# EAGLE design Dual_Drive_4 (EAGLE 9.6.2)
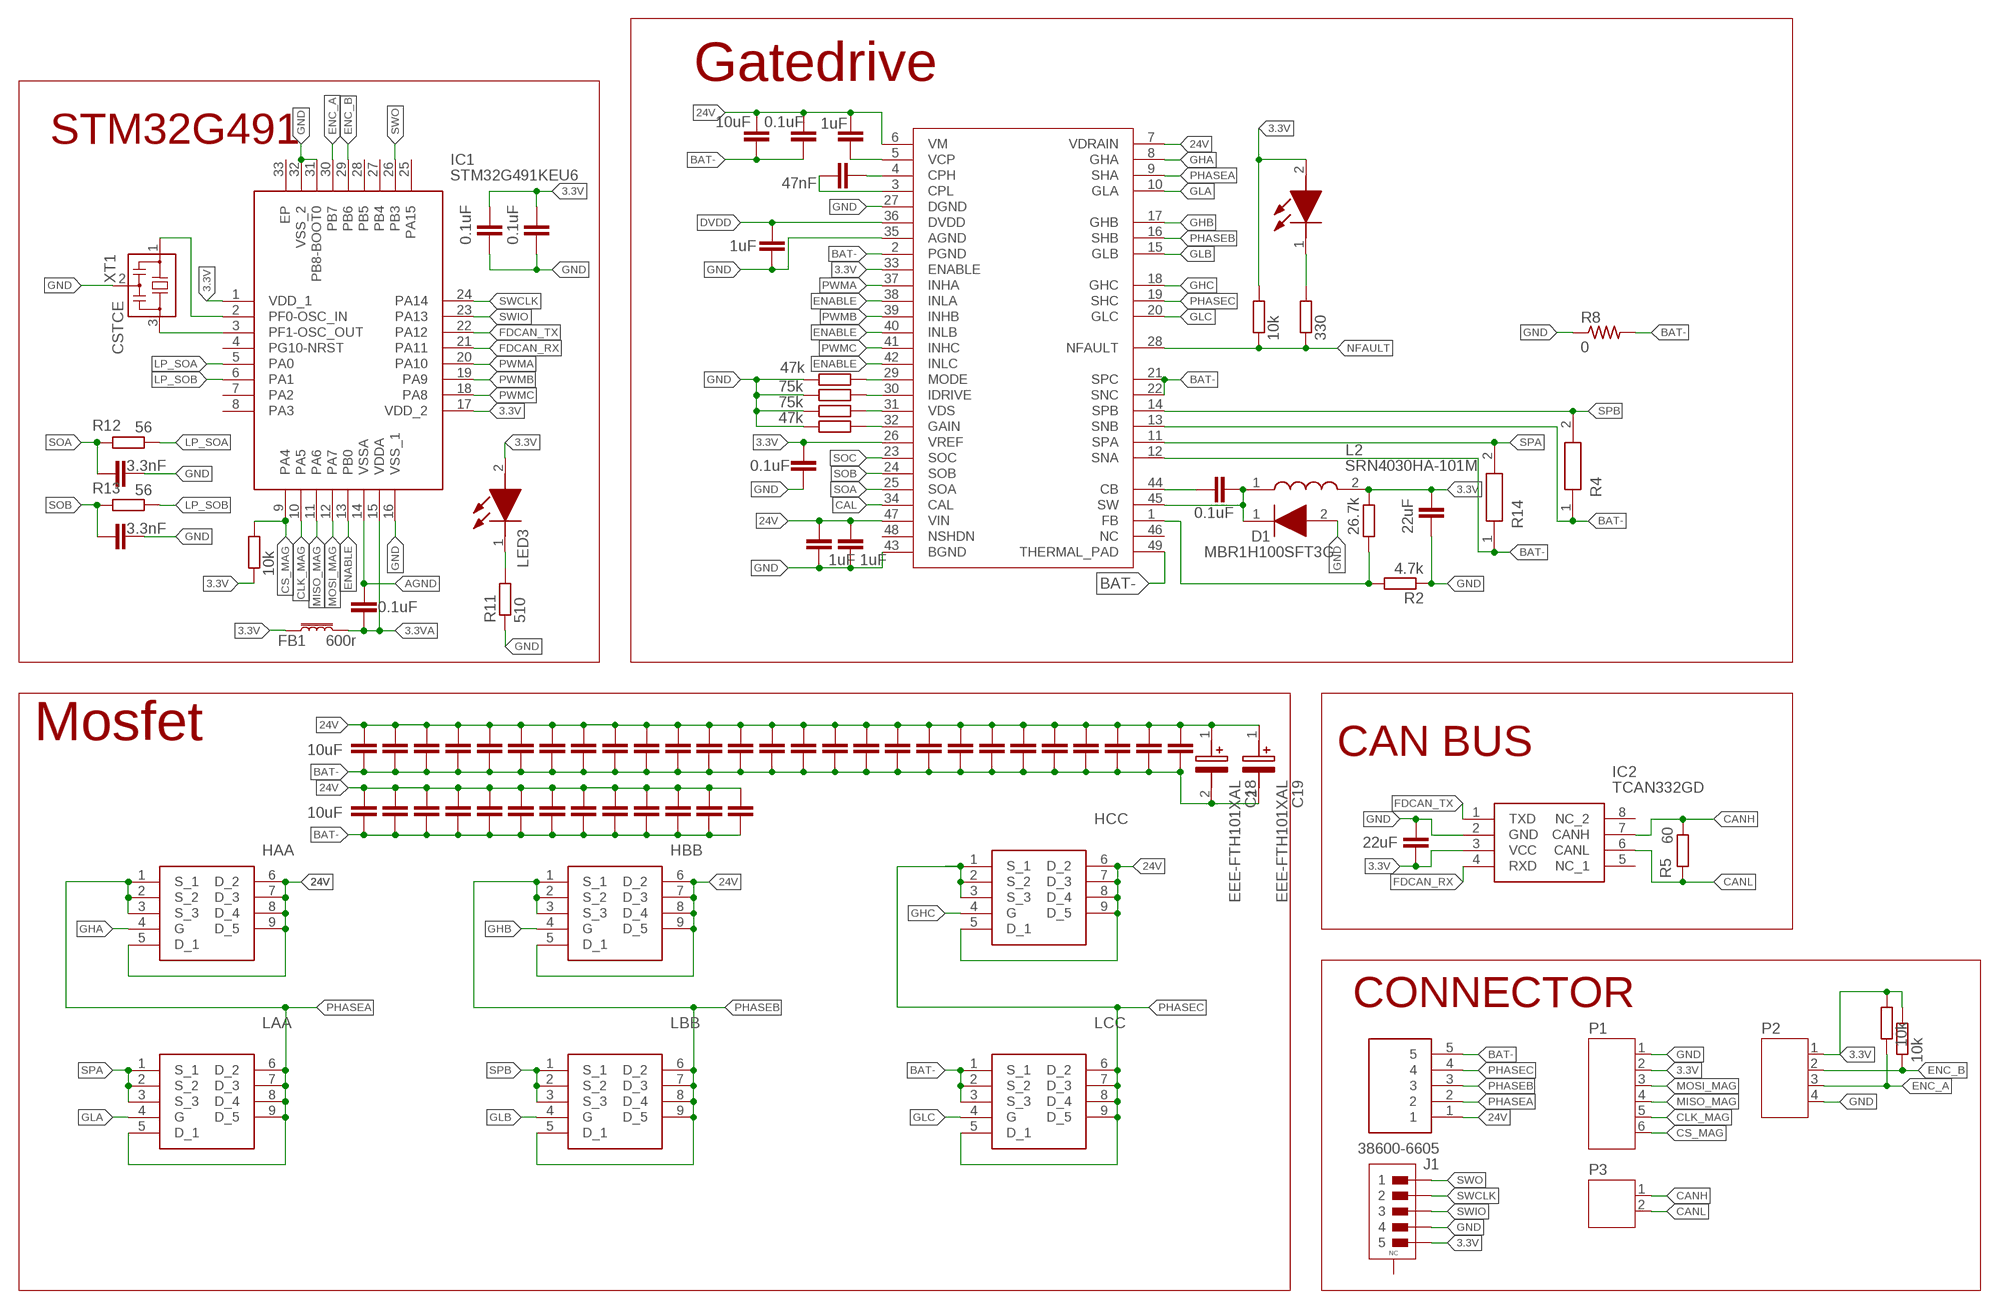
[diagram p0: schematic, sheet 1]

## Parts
C1  3.3nF  C-EUC0603  [C0603]
C2  3.3nF  C-EUC0603  [C0603]
C3  10uF  C-EU1206C1206  [C1206]
C4  22uF  C-EUC0603  [C0603]
C5  10uF  C-EU1206C1206  [C1206]
C6  10uF  C-EU1206C1206  [C1206]
C7  10uF  C-EU1206C1206  [C1206]
C8  10uF  C-EU1206C1206  [C1206]
C9  10uF  C-EU1206C1206  [C1206]
C10  0.1uF  C-EU1206C1206  [C1206]
C11  1uF  C-EUC0603  [C0603]
C12  10uF  C-EU1206C1206  [C1206]
C13  0.1uF  C-EUC0603  [C0603]
C14  1uF  C-EUC0603  [C0603]
C15  0.1uF  C-EUC0603  [C0603]
C16  10uF  C-EU1206C1206  [C1206]
C17  10uF  C-EU1206C1206  [C1206]
C18  EEE-FTH101XAL  [EEEHP1H4R7P]
C19  EEE-FTH101XAL  [EEEHP1H4R7P]
C20  10uF  C-EU1206C1206  [C1206]
C21  10uF  C-EU1206C1206  [C1206]
C22  10uF  C-EU1206C1206  [C1206]
C23  10uF  C-EU1206C1206  [C1206]
C24  10uF  C-EU1206C1206  [C1206]
C25  10uF  C-EU1206C1206  [C1206]
C26  0.1uF  C-EUC0603  [C0603]
C27  0.1uF  C-EUC0603  [C0603]
C28  10uF  C-EU1206C1206  [C1206]
C29  10uF  C-EU1206C1206  [C1206]
C30  0.1uF  C-EUC0603  [C0603]
C31  10uF  C-EU1206C1206  [C1206]
C32  10uF  C-EU1206C1206  [C1206]
C33  10uF  C-EU1206C1206  [C1206]
C34  10uF  C-EU1206C1206  [C1206]
C35  10uF  C-EU1206C1206  [C1206]
C36  10uF  C-EU1206C1206  [C1206]
C37  10uF  C-EU1206C1206  [C1206]
C38  10uF  C-EU1206C1206  [C1206]
C39  10uF  C-EU1206C1206  [C1206]
C40  10uF  C-EU1206C1206  [C1206]
C41  10uF  C-EU1206C1206  [C1206]
C42  10uF  C-EU1206C1206  [C1206]
C43  10uF  C-EU1206C1206  [C1206]
C44  10uF  C-EU1206C1206  [C1206]
C45  47nF  C-EU0805C0805  [C0805]
C46  22uF  C-EUC0603  [C0603]
C47  10uF  C-EU1206C1206  [C1206]
C48  10uF  C-EU1206C1206  [C1206]
C49  10uF  C-EU1206C1206  [C1206]
C50  10uF  C-EU1206C1206  [C1206]
C51  10uF  C-EU1206C1206  [C1206]
C52  10uF  C-EU1206C1206  [C1206]
C53  10uF  C-EU1206C1206  [C1206]
C54  10uF  C-EU1206C1206  [C1206]
C55  10uF  C-EU1206C1206  [C1206]
C56  10uF  C-EU1206C1206  [C1206]
CIN  1uF  C-EUC0603  [C0603]
CIN1  1uF  C-EUC0603  [C0603]
D1  MBR1H100SFT3G  [SODFL3616X98N]
FB1  600r  FERRITE_BEAD-0603  [0603]
HAA  TPH2R506PL,L1Q  [TPHR9003NLL1Q]
HBB  TPH2R506PL,L1Q  [TPHR9003NLL1Q]
HCC  TPH2R506PL,L1Q  [TPHR9003NLL1Q]
IC1  STM32G491KEU6  [QFN50P500X500X60-33N]
IC2  TCAN332GD  [SOIC127P600X175-8N]
IC3  DRV8323RHRGZR  [QFN50P700X700X100-49N]
J1  38600-6605  [386006605]
L2  SRN4030HA-101M  [SRN4030HA101M]
LAA  TPH2R506PL,L1Q  [TPHR9003NLL1Q]
LBB  TPH2R506PL,L1Q  [TPHR9003NLL1Q]
LCC  TPH2R506PL,L1Q  [TPHR9003NLL1Q]
LED1  LTST-C191KRKT  [LEDC1608X55N]
LED3  LTST-C191KRKT  [LEDC1608X55N]
P1  JST-PH6  [JST-PH6]
P2  JST-PH4  [JST-PH4]
P3  JST-PH2  [JST-PH2]
R1  26.7k  R-EU_R0603  [R0603]
R2  4.7k  R-EU_R0603  [R0603]
R3  47k  R-EU_R0603  [R0603]
R4  0.01  CRA2512-FZ-R010ELF  [RESC6434X90N]
R5  60  R-EU_R0603  [R0603]
R6  47k  R-EU_R0603  [R0603]
R7  75k  R-EU_R0603  [R0603]
R8  0  R-US_M1206  [M1206]
R10  75k  R-EU_R0603  [R0603]
R11  510  R-EU_R0603  [R0603]
R12  56  R-EU_R0603  [R0603]
R13  56  R-EU_R0603  [R0603]
R14  0.01  CRA2512-FZ-R010ELF  [RESC6434X90N]
RPULL  10k  R-EU_R0603  [R0603]
RPULL1  330  R-EU_R0603  [R0603]
RPULL2  10k  R-EU_R0603  [R0603]
RPULL3  10k  R-EU_R0603  [R0603]
RPULL4  10k  R-EU_R0603  [R0603]
U$3  CON-JST-PH2.0-5PIN-SMD  [CON-JST-PH2.0-5PIN-SMD]
XT1  CSTCE  [CSTCE]

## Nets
3.3V: C4.2 C15.1 C26.1 C27.1 C46.1 FB1.1 IC1.1(VDD_1) IC1.17(VDD_2) IC2.3(VCC) IC3.26(VREF) IC3.33(ENABLE) L2.2 LED1.2(A) LED3.2(A) P1.2 P2.1 R1.2 RPULL2.1 RPULL3.2 RPULL4.2 RPULL.2 U$3.5
3.3VA: C30.1 FB1.2 IC1.15(VDDA)
24V: C3.1 C5.1 C6.1 C7.1 C8.1 C9.1 C10.1 C11.1 C12.1 C16.1 C17.1 C18.1(+) C19.1(+) C20.1 C21.1 C22.1 C23.1 C24.1 C25.1 C28.1 C29.1 C31.1 C32.1 C33.1 C34.1 C35.1 C36.1 C37.1 C38.1 C39.1 C40.1 C41.1 C42.1 C43.1 C44.1 C47.1 C48.1 C49.1 C50.1 C51.1 C52.1 C53.1 C54.1 C55.1 C56.1 CIN1.1 CIN.1 HAA.5(D_1) HAA.6(D_2) HAA.7(D_3) HAA.8(D_4) HAA.9(D_5) HBB.5(D_1) HBB.6(D_2) HBB.7(D_3) HBB.8(D_4) HBB.9(D_5) HCC.5(D_1) HCC.6(D_2) HCC.7(D_3) HCC.8(D_4) HCC.9(D_5) IC3.6(VM) IC3.7(VDRAIN) IC3.47(VIN) J1.1
AGND: C30.2 IC1.14(VSSA)
BAT-: C3.2 C5.2 C6.2 C7.2 C8.2 C9.2 C10.2 C12.2 C16.2 C17.2 C18.2(-) C19.2(-) C20.2 C21.2 C22.2 C23.2 C24.2 C25.2 C28.2 C29.2 C31.2 C32.2 C33.2 C34.2 C35.2 C36.2 C37.2 C38.2 C39.2 C40.2 C41.2 C42.2 C43.2 C44.2 C47.2 C48.2 C49.2 C50.2 C51.2 C52.2 C53.2 C54.2 C55.2 C56.2 IC3.2(PGND) IC3.12(SNA) IC3.13(SNB) IC3.21(SPC) IC3.22(SNC) IC3.49(THERMAL_PAD) J1.5 LCC.1(S_1) LCC.2(S_2) LCC.3(S_3) R4.1 R8.2 R14.1
CAL: IC3.34(CAL)
CANH: IC2.7(CANH) P3.1 R5.1
CANL: IC2.6(CANL) P3.2 R5.2
CB: C13.1 IC3.44(CB)
CLK_MAG: IC1.10(PA5) P1.5
CPH: C45.2 IC3.4(CPH)
CPL: C45.1 IC3.3(CPL)
CS_MAG: IC1.9(PA4) P1.6 RPULL2.2
DVDD: C14.1 IC3.36(DVDD)
ENABLE: IC1.13(PB0) IC3.38(INLA) IC3.40(INLB) IC3.42(INLC)
ENC_A: IC1.30(PB7) P2.3 RPULL4.1
ENC_B: IC1.29(PB6) P2.2 RPULL3.1
FB: IC3.1(FB) R1.1 R2.2
FDCAN_RX: IC1.21(PA11) IC2.4(RXD)
FDCAN_TX: IC1.22(PA12) IC2.1(TXD)
GAIN: IC3.32(GAIN) R3.2
GHA: HAA.4(G) IC3.8(GHA)
GHB: HBB.4(G) IC3.17(GHB)
GHC: HCC.4(G) IC3.18(GHC)
GLA: IC3.10(GLA) LAA.4(G)
GLB: IC3.15(GLB) LBB.4(G)
GLC: IC3.20(GLC) LCC.4(G)
GND: C1.2 C2.2 C4.1 C14.2 C15.2 C26.2 C27.2 C46.2 CIN1.2 CIN.2 D1.2(A) IC1.16(VSS_1) IC1.31(PB8-BOOT0) IC1.32(VSS_2) IC2.2(GND) IC3.27(DGND) IC3.35(AGND) IC3.43(BGND) P1.1 P2.4 R2.1 R3.1 R6.1 R7.1 R8.1 R10.1 R11.1 U$3.4 XT1.2
IDRIVE: IC3.30(IDRIVE) R7.2
LEDFAULT: LED1.1(K) RPULL1.2
LP_SOA: IC1.5(PA0) R12.1
LP_SOB: IC1.6(PA1) R13.1
MISO_MAG: IC1.11(PA6) P1.4
MODE: IC3.29(MODE) R6.2
MOSI_MAG: IC1.12(PA7) P1.3
N$9: IC1.3(PF1-OSC_OUT) XT1.3
N$10: LED3.1(K) R11.2
N$11: IC1.2(PF0-OSC_IN) XT1.1
NFAULT: IC3.28(NFAULT) RPULL1.1 RPULL.1
PHASEA: HAA.1(S_1) HAA.2(S_2) HAA.3(S_3) IC3.9(SHA) J1.2 LAA.5(D_1) LAA.6(D_2) LAA.7(D_3) LAA.8(D_4) LAA.9(D_5)
PHASEB: HBB.1(S_1) HBB.2(S_2) HBB.3(S_3) IC3.16(SHB) J1.3 LBB.5(D_1) LBB.6(D_2) LBB.7(D_3) LBB.8(D_4) LBB.9(D_5)
PHASEC: HCC.1(S_1) HCC.2(S_2) HCC.3(S_3) IC3.19(SHC) J1.4 LCC.5(D_1) LCC.6(D_2) LCC.7(D_3) LCC.8(D_4) LCC.9(D_5)
PWMA: IC1.20(PA10) IC3.37(INHA)
PWMB: IC1.19(PA9) IC3.39(INHB)
PWMC: IC1.18(PA8) IC3.41(INHC)
SOA: C1.1 IC3.25(SOA) R12.2
SOB: C2.1 IC3.24(SOB) R13.2
SOC: IC3.23(SOC)
SPA: IC3.11(SPA) LAA.1(S_1) LAA.2(S_2) LAA.3(S_3) R14.2
SPB: IC3.14(SPB) LBB.1(S_1) LBB.2(S_2) LBB.3(S_3) R4.2
SW: C13.2 D1.1(K) IC3.45(SW) L2.1
SWCLK: IC1.24(PA14) U$3.2
SWIO: IC1.23(PA13) U$3.3
SWO: IC1.26(PB3) U$3.1
VCP: C11.2 IC3.5(VCP)
VDS: IC3.31(VDS) R10.2
Unconnected: IC1.4(PG10-NRST) IC1.7(PA2) IC1.8(PA3) IC1.25(PA15) IC1.27(PB4) IC1.28(PB5) IC1.33(EP) IC2.5(NC_1) IC2.8(NC_2) IC3.46(NC) IC3.48(NSHDN) U$3.NC1(NC) U$3.NC2(NC)

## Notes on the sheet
- Gatedrive
- STM32G491
- Mosfet
- CAN BUS
- CONNECTOR

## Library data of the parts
C1 C2 C26 C27 C30 = rcl:C-EU: CAPACITOR, European symbol; SPICEPREFIX: C
C3 C5-C10 C12 C16 C17 C20-C25 C28 C29 C31-C44 C47-C56 = projectieie:C-EU1206: CAPACITOR, European symbol; SPICEPREFIX: C
C4 C11 C13-C15 C46 CIN CIN1 = projectieie:C-EU: CAPACITOR, European symbol; SPICEPREFIX: C
C18 C19 = EEE-FTH101XAL:EEE-FTH101XAL: Aluminum Electrolytic Capacitors - SMD 50VDC 100uF 20% 6x8mm AEC-Q200; DESCRIPTION: Aluminum Electrolytic Capacitors - SMD 50VDC 100uF 20% 6x8mm AEC-Q200; HEIGHT: mm; MANUFACTURER_NAME: Panasonic; MANUFACTURER_PART_NUMBER: EEE-FTH101XAL; MOUSER_PART_NUMBER: 667-EEE-FTH101XAL; MOUSER_PRICE-STOCK: https://www.mouser.co.uk/ProductDetail/Panasonic/EEE-FTH101XAL?qs=vmHwEFxEFR%252BNutcOP%252Bqsmw%3D%3D
C45 = projectieie:C-EU0805: CAPACITOR, European symbol; SPICEPREFIX: C
D1 = MBR1H100SFT3G:MBR1H100SFT3G: Diode Schottky 100V 1A SOD123FL ON Semiconductor MBR1H100SFT3G Schottky Diode, 1A, 100V, 2-Pin SOD-123FL; ARROW_PART_NUMBER: MBR1H100SFT3G; ARROW_PRICE-STOCK: https://www.arrow.com/en/products/mbr1h100sft3g/on-semiconductor; DESCRIPTION: Diode Schottky 100V 1A SOD123FL ON Semiconductor MBR1H100SFT3G Schottky Diode, 1A, 100V, 2-Pin SOD-123FL; HEIGHT: 0.98mm; MANUFACTURER_NAME: ON Semiconductor; MANUFACTURER_PART_NUMBER: MBR1H100SFT3G; MOUSER_PART_NUMBER: 863-MBR1H100SFT3G; MOUSER_PRICE-STOCK: https://www.mouser.co.uk/ProductDetail/ON-Semiconductor/MBR1H100SFT3G?qs=0n%252BW%2FEG%252BKm6mjS2tdY4y%2FA%3D%3D
FB1 = SparkFun-Coils:FERRITE_BEAD: Ferrite Bead (blocks, cores, rings, chokes, etc.); PROD_ID: NDUC-13805; VALUE: 30Ω/1.8A
HAA HBB HCC LAA LBB LCC = TPH2R506PL_L1Q:TPH2R506PL,L1Q: MOSFET N-Ch 60V 4180pF 60nC 160A 132W Source: Datasheet; ARROW_PART_NUMBER: TPH2R506PL,L1Q; ARROW_PRICE-STOCK: https://www.arrow.com/en/products/tph2r506pll1q/toshiba; DESCRIPTION: MOSFET N-Ch 60V 4180pF 60nC 160A 132W; HEIGHT: 1mm; MANUFACTURER_NAME: Toshiba; MANUFACTURER_PART_NUMBER: TPH2R506PL,L1Q; MOUSER_PART_NUMBER: 757-TPH2R506PLL1Q; MOUSER_PRICE-STOCK: https://www.mouser.co.uk/ProductDetail/Toshiba/TPH2R506PLL1Q?qs=bUPhaerQQeFGJjj6SxbPEQ%3D%3D
IC1 = STM32G491KEU6:STM32G491KEU6: MCU 32-bit ARM Cortex M4 RISC 512KB Flash 1.8V/2.5V/3.3V 32-Pin UFQFPN EP Tray Source: Datasheet; ARROW_PART_NUMBER: STM32G491KEU6; ARROW_PRICE-STOCK: https://www.arrow.com/en/products/stm32g491keu6/stmicroelectronics?region=nac; DESCRIPTION: MCU 32-bit ARM Cortex M4 RISC 512KB Flash 1.8V/2.5V/3.3V 32-Pin UFQFPN EP Tray; HEIGHT: 0.6mm; MANUFACTURER_NAME: STMicroelectronics; MANUFACTURER_PART_NUMBER: STM32G491KEU6; MOUSER_PART_NUMBER: 511-STM32G491KEU6; MOUSER_PRICE-STOCK: https://www.mouser.co.uk/ProductDetail/STMicroelectronics/STM32G491KEU6?qs=eP2BKZSCXI6Ifx0U7HNJyA%3D%3D
IC2 = TCAN332GD:TCAN332GD: 3.3-V CAN Transceivers with CAN FD (Flexible Data Rate) Source: Datasheet; ARROW_PART_NUMBER: TCAN332GD; ARROW_PRICE-STOCK: https://www.arrow.com/en/products/tcan332gd/texas-instruments?region=nac; DESCRIPTION: 3.3-V CAN Transceivers with CAN FD (Flexible Data Rate); HEIGHT: 1.75mm; MANUFACTURER_NAME: Texas Instruments; MANUFACTURER_PART_NUMBER: TCAN332GD; MOUSER_PART_NUMBER: 595-TCAN332GD; MOUSER_PRICE-STOCK: https://www.mouser.co.uk/ProductDetail/Texas-Instruments/TCAN332GD?qs=n%252BTO0c4TDSYoXh39%2FoLTXQ%3D%3D
IC3 = projectieie:DRV8323RHRGZR: 60V Three-Phase Smart Gate Driver With Buck Regulator and Three Current Shunt Amplifiers Source: Datasheet; ARROW_PART_NUMBER: DRV8323RHRGZR; ARROW_PRICE-STOCK: https://www.arrow.com/en/products/drv8323rhrgzr/texas-instruments; DESCRIPTION: 60V Three-Phase Smart Gate Driver With Buck Regulator and Three Current Shunt Amplifiers; HEIGHT: 1mm; MANUFACTURER_NAME: Texas Instruments; MANUFACTURER_PART_NUMBER: DRV8323RHRGZR; MOUSER_PART_NUMBER: 595-DRV8323RHRGZR; MOUSER_PRICE-STOCK: https://www.mouser.co.uk/ProductDetail/Texas-Instruments/DRV8323RHRGZR?qs=Mv7BduZupUj%2FALPfD5cVcg%3D%3D
J1 = 38600-6605:38600-6605: Barrier Terminal Blocks SR BTS CS PC 5ASYCP Source: Datasheet; DESCRIPTION: Barrier Terminal Blocks SR BTS CS PC 5ASYCP; HEIGHT: 12.7mm; MANUFACTURER_NAME: Molex; MANUFACTURER_PART_NUMBER: 38600-6605; MOUSER_PART_NUMBER: 538-38600-6605; MOUSER_PRICE-STOCK: https://www.mouser.com/Search/Refine.aspx?Keyword=538-38600-6605
L2 = SRN4030HA-101M:SRN4030HA-101M: Ind,4x4x3mm,100uH+/-20%,0.55A,150C,shd; DESCRIPTION: Ind,4x4x3mm,100uH+/-20%,0.55A,150C,shd; HEIGHT: 3mm; MANUFACTURER_NAME: Bourns; MANUFACTURER_PART_NUMBER: SRN4030HA-101M
LED1 LED3 = LTST-C191KRKT:LTST-C191KRKT: Standard LEDs - SMD Red Clear 631nm; ARROW_PART_NUMBER: LTST-C191KRKT; ARROW_PRICE-STOCK: https://www.arrow.com/en/products/ltst-c191krkt/lite-on-technology; DESCRIPTION: Standard LEDs - SMD Red Clear 631nm; HEIGHT: 0.55mm; MANUFACTURER_NAME: Lite-On; MANUFACTURER_PART_NUMBER: LTST-C191KRKT; MOUSER_PART_NUMBER: 859-LTST-C191KRKT; MOUSER_PRICE-STOCK: https://www.mouser.co.uk/ProductDetail/Lite-On/LTST-C191KRKT?qs=BAIUz4Y8PJBLfOhzue0q%252BA%3D%3D
P1 = jst-ph:JST-PH6
P2 = jst-ph:JST-PH4
P3 = jst-ph:JST-PH2
R1 R2 RPULL RPULL1-RPULL4 = projectieie:R-EU_: RESISTOR, European symbol; SPICEPREFIX: R
R3 R5-R7 R10-R13 = rcl:R-EU_: RESISTOR, European symbol; SPICEPREFIX: R
R4 R14 = CRA2512-FZ-R010ELF:CRA2512-FZ-R010ELF: Bourns CRA Series High Power Surface Mount Resistor 2512 Case 10m +/-1% 3W +/-75ppm/C; ARROW_PART_NUMBER: CRA2512-FZ-R010ELF; ARROW_PRICE-STOCK: https://www.arrow.com/en/products/cra2512-fz-r010elf/bourns; DESCRIPTION: Bourns CRA Series High Power Surface Mount Resistor 2512 Case 10m +/-1% 3W +/-75ppm/C; HEIGHT: 0.9mm; MANUFACTURER_NAME: Bourns; MANUFACTURER_PART_NUMBER: CRA2512-FZ-R010ELF; MOUSER_PART_NUMBER: 652-CRA2512FZR010ELF; MOUSER_PRICE-STOCK: https://www.mouser.co.uk/ProductDetail/Bourns/CRA2512-FZ-R010ELF?qs=WqWCsLCZBkoNPiv%2FXVnYvw%3D%3D
R8 = rcl:R-US_: RESISTOR, American symbol; SPICEPREFIX: R
U$3 = con-jst-ph2.0:CON-JST-PH2.0-5PIN-SMD
XT1 = sc_usercreated:CSTCE

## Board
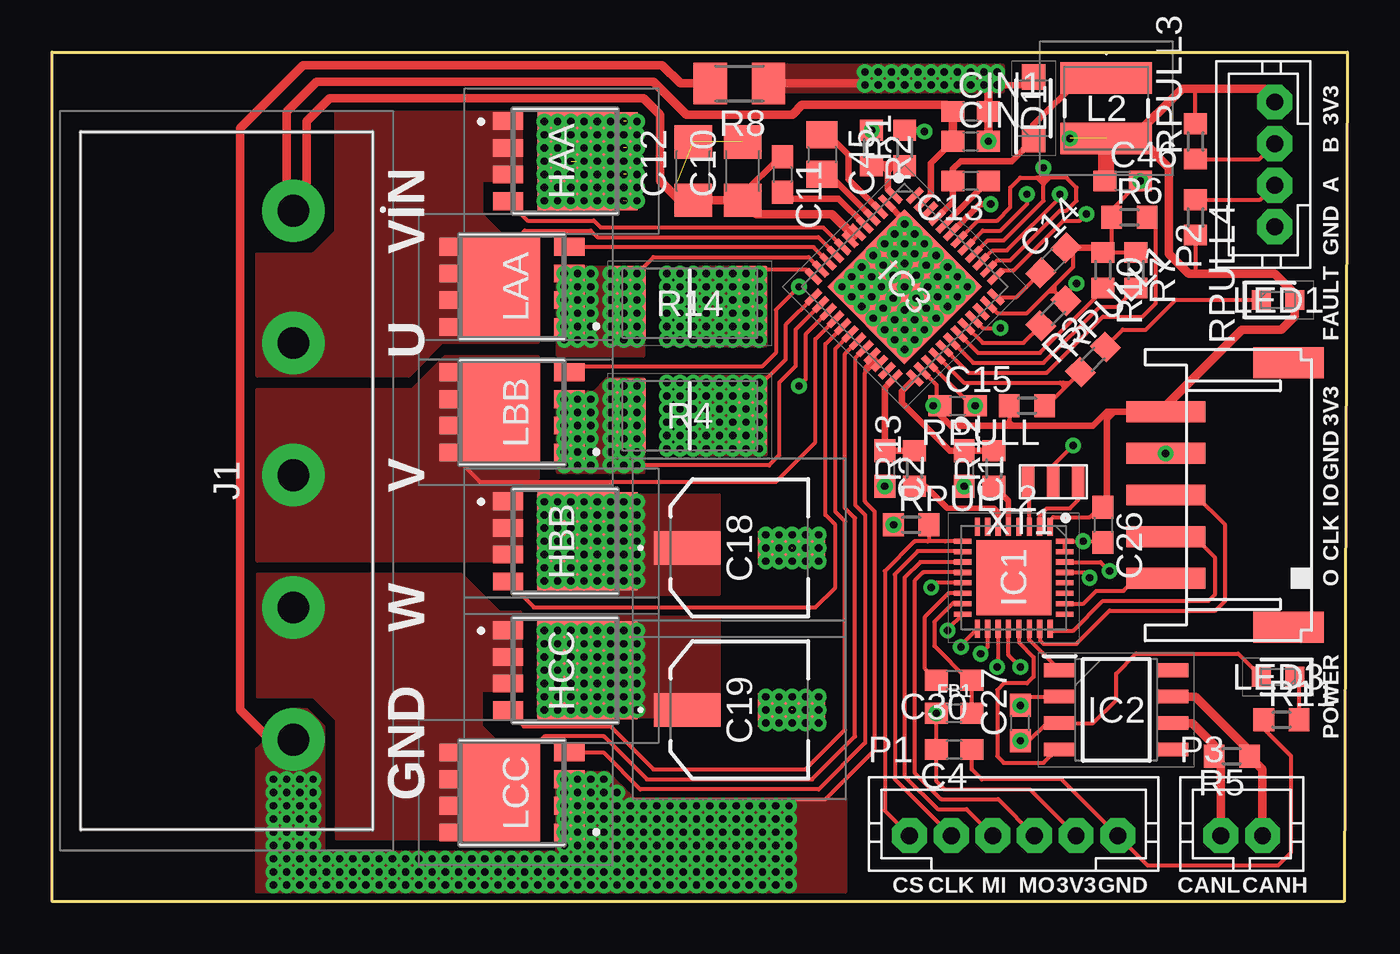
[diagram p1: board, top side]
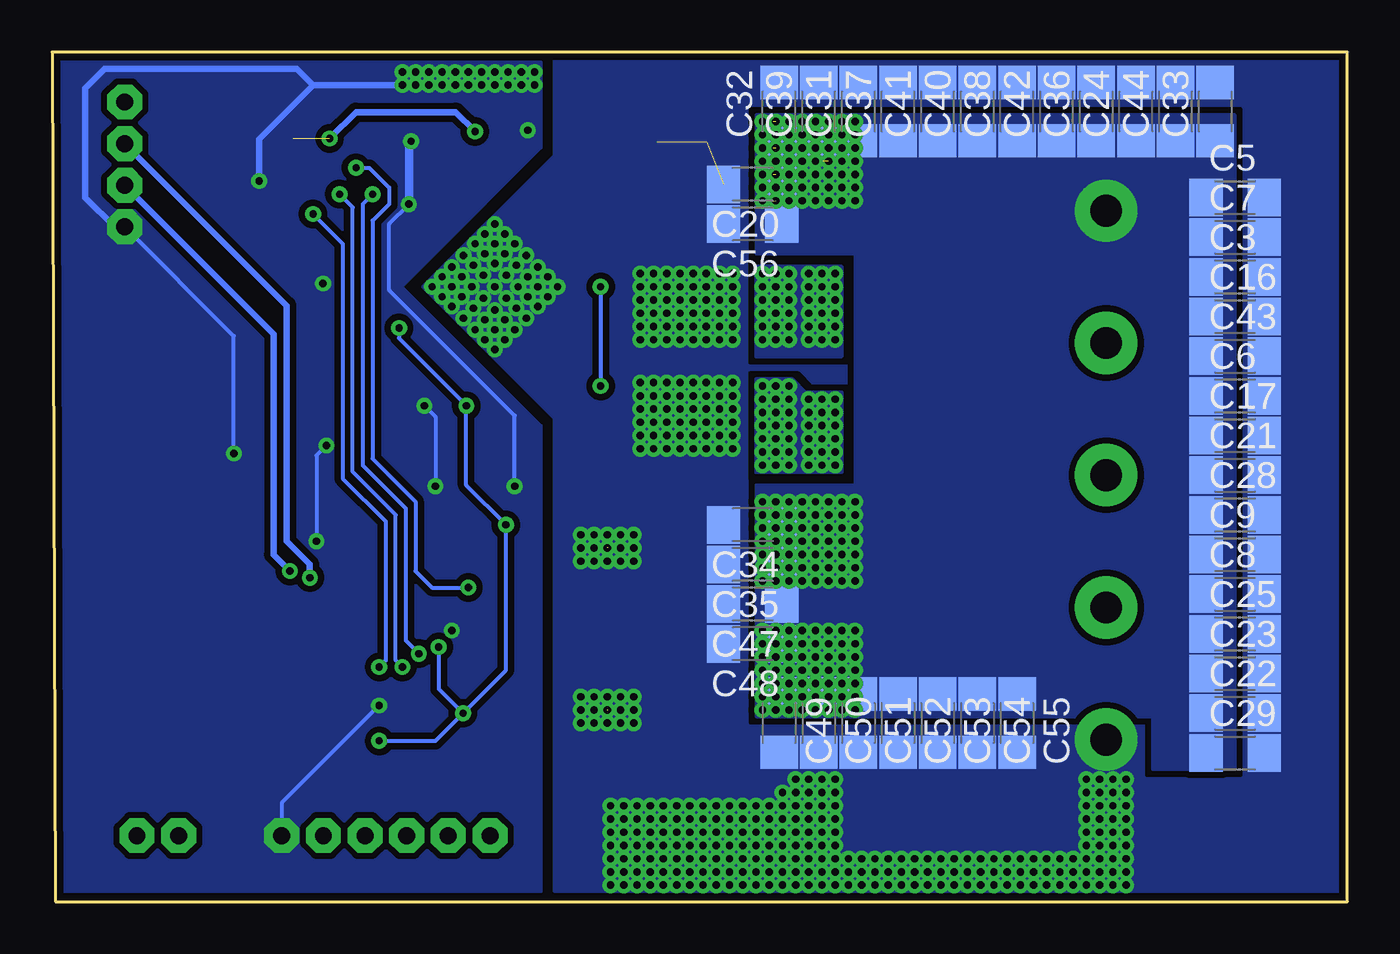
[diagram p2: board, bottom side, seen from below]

Size 62.23 x 40.8 mm. Coordinates in mm from the lower left corner, seen from the top.
Outline: 62.07,0 0,0 0,40.8 62.23,40.8 62.07,0
Copper layers (1*16): Top 0.035mm / dielectric 1.5mm / Bottom 0.035mm
Design rules "default *": minimum track width 6mil, minimum drill 0.35mm, track to track 6mil, track to pad 6mil, pad to pad 6mil, via to via 6mil, smd to smd 6mil, copper to edge 6mil, drill to drill 6mil, minimum pad ring 10mil, minimum via ring 8mil, stop-mask expansion 4mil, vias tented up to drill 15mil, thermal gap 10mil

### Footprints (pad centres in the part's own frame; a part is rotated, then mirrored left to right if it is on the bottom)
C0603 = smd 1.1 x 1: 1 -0.85,0; 2 0.85,0
C1206 = smd 1.6 x 1.8: 1 -1.4,0; 2 1.4,0
EEEHP1H4R7P = smd 1.6 x 3.2: 1 0,-2.5; 2 0,2.5
C0805 = smd 1.3 x 1.5: 1 -0.95,0; 2 0.95,0
SODFL3616X98N = smd 1.24 x 1.12: 1 -1.5,0; 2 1.5,0
0603 = smd 1.1 x 1: 1 -0.85,0; 2 0.85,0
TPHR9003NLL1Q = smd 0.85 x 1.45: 1 -1.925,-2.309; 2 -0.635,-2.309; 3 0.635,-2.309; 4 1.925,-2.309 | smd 0.85 x 1.05: 5 1.925,3.391; 6 0.635,3.391; 7 -0.635,3.391; 8 -1.925,3.391 | smd 4.7 x 3.75: 9 0,0.981
QFN50P500X500X60-33N = smd 0.85 x 0.25: 1 -2.45,1.75; 2 -2.45,1.25; 3 -2.45,0.75; 4 -2.45,0.25; 5 -2.45,-0.25; 6 -2.45,-0.75; 7 -2.45,-1.25; 8 -2.45,-1.75; 17 2.45,-1.75; 18 2.45,-1.25; 19 2.45,-0.75; 20 2.45,-0.25; 21 2.45,0.25; 22 2.45,0.75; 23 2.45,1.25; 24 2.45,1.75 | smd 0.25 x 0.85: 9 -1.75,-2.45; 10 -1.25,-2.45; 11 -0.75,-2.45; 12 -0.25,-2.45; 13 0.25,-2.45; 14 0.75,-2.45; 15 1.25,-2.45; 16 1.75,-2.45; 25 1.75,2.45; 26 1.25,2.45; 27 0.75,2.45; 28 0.25,2.45; 29 -0.25,2.45; 30 -0.75,2.45; 31 -1.25,2.45; 32 -1.75,2.45 | smd 3.6 x 3.6: 33 0,0
SOIC127P600X175-8N = smd 1.528 x 0.65: 1 -2.711,1.905; 2 -2.711,0.635; 3 -2.711,-0.635; 4 -2.711,-1.905; 5 2.711,-1.905; 6 2.711,-0.635; 7 2.711,0.635; 8 2.711,1.905
QFN50P700X700X100-49N = smd 0.9 x 0.3: 1 -3.45,2.75; 2 -3.45,2.25; 3 -3.45,1.75; 4 -3.45,1.25; 5 -3.45,0.75; 6 -3.45,0.25; 7 -3.45,-0.25; 8 -3.45,-0.75; 9 -3.45,-1.25; 10 -3.45,-1.75; 11 -3.45,-2.25; 12 -3.45,-2.75; 25 3.45,-2.75; 26 3.45,-2.25; 27 3.45,-1.75; 28 3.45,-1.25; 29 3.45,-0.75; 30 3.45,-0.25; 31 3.45,0.25; 32 3.45,0.75; 33 3.45,1.25; 34 3.45,1.75; 35 3.45,2.25; 36 3.45,2.75 | smd 0.3 x 0.9: 13 -2.75,-3.45; 14 -2.25,-3.45; 15 -1.75,-3.45; 16 -1.25,-3.45; 17 -0.75,-3.45; 18 -0.25,-3.45; 19 0.25,-3.45; 20 0.75,-3.45; 21 1.25,-3.45; 22 1.75,-3.45; 23 2.25,-3.45; 24 2.75,-3.45; 37 2.75,3.45; 38 2.25,3.45; 39 1.75,3.45; 40 1.25,3.45; 41 0.75,3.45; 42 0.25,3.45; 43 -0.25,3.45; 44 -0.75,3.45; 45 -1.25,3.45; 46 -1.75,3.45; 47 -2.25,3.45; 48 -2.75,3.45 | smd 5.25 x 5.25: 49 0,0
386006605 = drill 1.524 pad 3: 1 0,0; 2 6.35,0; 3 12.7,0; 4 19.05,0; 5 25.4,0
SRN4030HA101M = smd 4.4 x 1.5: 1 0,-1.45; 2 0,1.45
LEDC1608X55N = smd 0.9 x 0.95: 1 -0.8,0; 2 0.8,0
JST-PH6 = drill 0.813 pad 1.676 octagon: 1 5,0; 2 3,0; 3 1,0; 4 -1,0; 5 -3,0; 6 -5,0
JST-PH4 = drill 0.813 pad 1.676 octagon: 1 3,0; 2 1,0; 3 -1,0; 4 -3,0
JST-PH2 = drill 0.813 pad 1.676 octagon: 1 1,0; 2 -1,0
R0603 = smd 1 x 1.1: 1 -0.85,0; 2 0.85,0
RESC6434X90N = smd 1.55 x 3.55: 1 -2.9,0; 2 2.9,0
M1206 = smd 1.6 x 2: 1 -1.4,0; 2 1.4,0
CON-JST-PH2.0-5PIN-SMD = smd 1 x 3.8: 1 4,0; 2 2,0; 3 0,0; 4 -2,0; 5 -4,0 | smd 1.5 x 3.4: NC1 -6.35,5.9; NC2 6.35,5.9
CSTCE = smd 0.6 x 1.6: 1 -1.2,0; 2 0,0; 3 1.2,0

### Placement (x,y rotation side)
C1  43.81,20.8 270 top
C2  40.01,20.8 270 top
C3  5.4,30 0 bottom
C4  43.34,7.3 180 top
C5  5.4,33.81 0 bottom
C6  5.4,24.29 0 bottom
C7  5.4,31.91 0 bottom
C8  5.4,14.76 0 bottom
C9  5.4,16.67 0 bottom
C10  33.18,35.08 90 top
C11  35.08,34.92 270 top
C12  30.8,35.08 90 top
C13  44.13,34.61 180 top
C14  48.1,30.8 45 top
C15  43.5,23.81 0 top
C16  5.4,28.1 0 bottom
C17  5.4,22.38 0 bottom
C18  33.02,16.99 270 top
C19  33.02,9.21 270 top
C20  28.57,34.45 180 bottom
C21  5.4,20.48 0 bottom
C22  5.4,9.05 0 bottom
C23  5.4,10.95 0 bottom
C24  10.16,37.94 90 bottom
C25  5.4,12.86 0 bottom
C26  50.48,18.1 270 top
C27  46.51,8.57 90 top
C28  5.4,18.57 0 bottom
C29  5.4,7.14 0 bottom
C30  43.34,10.64 180 top
C31  23.5,37.94 90 bottom
C32  27.3,37.94 90 bottom
C33  6.35,37.94 90 bottom
C34  28.57,18.1 180 bottom
C35  28.57,16.19 180 bottom
C36  12.06,37.94 90 bottom
C37  21.59,37.94 90 bottom
C38  15.88,37.94 90 bottom
C39  25.4,37.94 90 bottom
C40  17.78,37.94 90 bottom
C41  19.68,37.94 90 bottom
C42  13.97,37.94 90 bottom
C43  5.4,26.19 0 bottom
C44  8.26,37.94 90 bottom
C45  36.99,35.88 270 top
C46  51.44,34.61 0 top
C47  28.57,14.29 180 bottom
C48  28.57,12.38 180 bottom
C49  27.3,8.57 270 bottom
C50  25.4,8.57 270 bottom
C51  23.5,8.57 270 bottom
C52  21.59,8.57 270 bottom
C53  19.68,8.57 270 bottom
C54  17.78,8.57 270 bottom
C55  15.88,8.57 270 bottom
C56  28.57,32.54 180 bottom
CIN  44.13,36.51 0 top
CIN1  44.13,37.94 0 top
D1  47.15,38.1 90 top
FB1  43.34,9.05 0 top
HAA  24.21,35.56 270 top
HBB  24.21,17.3 270 top
HCC  24.21,11.11 270 top
IC1  46.2,15.56 270 top
IC2  51.12,9.21 0 top
IC3  40.96,29.53 315 top
J1  11.59,33.18 270 top
L2  50.64,38.1 180 top
LAA  22.54,29.53 90 top
LBB  22.54,23.5 90 top
LCC  22.54,5.24 90 top
LED1  58.9,28.89 0 top
LED3  58.9,10.79 180 top
P1  46.2,3.17 0 top
P2  58.74,35.4 90 top
P3  57.15,3.17 0 top
R1  40.96,36.2 90 top
R2  39.37,36.2 270 top
R3  48.1,28.26 225 top
R4  30.64,23.34 180 top
R5  56.67,6.99 180 top
R6  51.75,32.86 0 top
R7  52.07,30.32 270 top
R8  33.02,39.29 180 top
R10  50.48,30.32 270 top
R11  59.05,8.73 0 top
R12  45.24,20.8 90 top
R13  41.43,20.8 90 top
R14  30.64,28.73 180 top
RPULL  46.83,23.81 180 top
RPULL1  50.01,26.04 45 top
RPULL2  41.27,18.1 0 top
RPULL3  54.93,36.51 90 top
RPULL4  54.93,32.86 270 top
U$3  53.5,19.53 270 top
XT1  48.1,20.16 180 top

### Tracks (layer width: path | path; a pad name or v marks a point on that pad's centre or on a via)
3.3V  (via drill 0.35)  (1 unrouted)
  Top 0.203: IC3.33 44.71,27.54 v45.56,27.54 | IC3.26 42.49,24.81 42.49,23.97 v42.33,23.81 42.33,23.71 43.18,22.86 45.72,22.86 | 45.72,22.86 46.2,22.86 | RPULL.2 45.98,23.12 | 45.98,23.12 45.72,22.86 | 45.98,23.12 45.98,23.07 46.2,22.86 | IC1.1 47.95,18.32 48.09,18.47 49.85,18.47 50.22,18.84 50.32,18.95 | 50.16,18.95 50.32,18.95 | 50.32,18.95 C26.1 | P1.2 46.97,5.4 42.86,5.4 42.49,5.77 C4.2 FB1.1 | C27.1 46.93,7.72 47.78,8.57 IC2.3 50.01,8.57 51.12,9.68 51.12,10.95 52.07,11.91 56.98,11.91 LED3.2 | 50.01,22.86 46.2,22.86 | 53.85,23.53 U$3.5 | IC1.17 43.66,12.32 v43.66,12.22 | RPULL3.2 54.93,39.04 | RPULL4.2 54.93,30.16
  Top 0.305: R1.2 41.85,37.05 v41.91,36.99 | U$3.5 51.02,23.53 | 51.02,23.53 50.67,23.53 | 50.67,23.18 50.67,19.3 50.22,18.84 | 50.67,23.18 50.67,23.53 | 50.67,23.53 50.01,22.86 43.18,22.86 42.65,23.39 C15.1 | 50.67,23.18 51.02,23.53
  Top 0.406: P2.1 58.26,38.88 58.26,39.04 54.93,39.04 54.29,39.04 51.91,36.65 L2.2 52.25,36.65 53.66,35.24 53.66,31.11 54.61,30.16 54.93,30.16 58.74,30.16 59.7,29.2 LED1.2 59.7,28.11 59.05,27.46 57.15,27.46 53.5,23.81 U$3.5
  Top 0.762: C46.1 50.64,34.66 L2.2
  Bottom 0.203: FB1.1 40.42,11.11 RPULL2.1 42.33,20 v42.33,23.81 42.33,23.84 45.56,27.07 v45.56,27.54 | C27.1 43.81,7.72 FB1.1 | v43.66,12.22 43.66,10.22 FB1.1
  Bottom 0.305: v41.91,36.99 42.84,37.92 47.62,37.92 v48.9,36.65
  other vias: 40.42,18.1 42.49,9.05 46.51,7.72
3.3VA
  Top 0.203: IC1.15 43.71,14.35 43.3,14.35 42.39,13.44 42.39,12.28 44.03,10.64 C30.1 FB1.2
24V  (via drill 0.35)  (5 unrouted)
  Top 0.203: C10.1 33.18,33.97 | C11.1 34.98,35.77
  Top 0.305: IC3.7 38.52,31.97 IC3.6 | 34.98,35.77 33.18,33.97 | IC3.47 42.23,33.98 42.23,35.46 CIN.1
  Top 0.406: 38.52,31.97 | 38.52,31.97 37.47,33.02 33.84,33.02 C10.1 C12.1 30.13,33.68 29.21,34.61 29.21,37.78 28.42,38.58 13.34,38.58 12.22,37.47 12.22,33.81 J1.1 11.27,33.5 11.27,37.94 12.7,39.37 28.89,39.37 30.48,37.78 35.56,37.78 36.04,38.26 42.97,38.26 CIN1.1 CIN.1
  other vias: 23.65,37.47 24.29,37.47 24.92,37.47 25.56,37.47 26.19,37.47 26.83,37.47 27.46,37.47 28.1,37.47 23.65,36.83 24.29,36.83 24.92,36.83 25.56,36.83 26.19,36.83 26.83,36.83 27.46,36.83 28.1,36.83 23.65,36.2 24.29,36.2 24.92,36.2 25.56,36.2 26.19,36.2 26.83,36.2 27.46,36.2 28.1,36.2 23.65,35.56 24.29,35.56 24.92,35.56 25.56,35.56 26.19,35.56 26.83,35.56 27.46,35.56 28.1,35.56 23.65,34.92 24.29,34.92 24.92,34.92 25.56,34.92 26.19,34.92 26.83,34.92 27.46,34.92 28.1,34.92 23.65,34.29 24.29,34.29 24.92,34.29 25.56,34.29 26.19,34.29 26.83,34.29 27.46,34.29 28.1,34.29 23.65,33.66 24.29,33.66 24.92,33.66 25.56,33.66 26.19,33.66 26.83,33.66 27.46,33.66 28.1,33.66 23.65,19.21 24.29,19.21 24.92,19.21 25.56,19.21 26.19,19.21 26.83,19.21 27.46,19.21 28.1,19.21 23.65,18.57 24.29,18.57 24.92,18.57 25.56,18.57 26.19,18.57 26.83,18.57 27.46,18.57 28.1,18.57 23.65,17.94 24.29,17.94 24.92,17.94 25.56,17.94 26.19,17.94 26.83,17.94 27.46,17.94 28.1,17.94 23.65,17.3 24.29,17.3 24.92,17.3 25.56,17.3 26.19,17.3 26.83,17.3 27.46,17.3 28.1,17.3 23.65,16.67 24.29,16.67 24.92,16.67 25.56,16.67 26.19,16.67 26.83,16.67 27.46,16.67 28.1,16.67 23.65,16.03 24.29,16.03 24.92,16.03 25.56,16.03 26.19,16.03 26.83,16.03 27.46,16.03 28.1,16.03 23.65,15.4 24.29,15.4 24.92,15.4 25.56,15.4 26.19,15.4 26.83,15.4 27.46,15.4 28.1,15.4 23.65,13.02 24.29,13.02 24.92,13.02 25.56,13.02 26.19,13.02 26.83,13.02 27.46,13.02 28.1,13.02 23.65,12.38 24.29,12.38 24.92,12.38 25.56,12.38 26.19,12.38 26.83,12.38 27.46,12.38 28.1,12.38 23.65,11.75 24.29,11.75 24.92,11.75 25.56,11.75 26.19,11.75 26.83,11.75 27.46,11.75 28.1,11.75 23.65,11.11 24.29,11.11 24.92,11.11 25.56,11.11 26.19,11.11 26.83,11.11 27.46,11.11 28.1,11.11 23.65,10.48 24.29,10.48 24.92,10.48 25.56,10.48 26.19,10.48 26.83,10.48 27.46,10.48 28.1,10.48 23.65,9.84 24.29,9.84 24.92,9.84 25.56,9.84 26.19,9.84 26.83,9.84 27.46,9.84 28.1,9.84 23.65,9.21 24.29,9.21 24.92,9.21 25.56,9.21 26.19,9.21 26.83,9.21 27.46,9.21 28.1,9.21
  pour Top (no thermals): 23.34,19.53 23.34,14.76 32.07,14.76 32.07,19.53
  pour Top (no thermals): 23.34,13.65 23.34,8.89 32.07,8.89 32.07,13.65
  pour Bottom (isolate 0.305, no thermals): 5.4,37.78 28.42,37.78 28.42,31.11 23.65,31.11 23.65,20 28.42,20 28.42,8.89 9.37,8.89 9.37,6.35 5.4,6.35
AGND
  Top 0.203: IC1.14 43.06,14.81 41.91,13.65 41.91,11.21 C30.2 42.33,10.79
BAT-  (via drill 0.35)  (4 unrouted)
  Top 0.203: IC3.12 36.26,30.34 33.99,30.34 33.54,29.89 R14.1 | IC3.13 35.24,27.7 35.24,26.04 33.54,24.33 R4.1 | v27.78,4.6 27.78,4.92 37.15,4.92 39.53,7.3 39.53,18.73 39.05,19.21 39.05,25.4 | IC3.21 39.51,26.1 | 39.51,26.1 IC3.22 39.5,25.85 39.05,25.4 | 39.51,26.1 39.05,25.64 39.05,25.4
  Top 0.305: IC3.2 40.96,32.71 v40.96,32.54 IC3.49
  Top 0.406: J1.5 10.48,7.78 9.05,9.21 9.05,37.15 12.06,40.16 29.31,40.16 30.19,39.29 R8.2
  other vias: 24.61,5.87 24.61,5.24 24.61,4.6 24.61,3.97 24.61,3.33 25.24,5.87 25.24,5.24 25.24,4.6 25.24,3.97 25.24,3.33 25.88,3.33 25.88,3.97 25.88,4.6 25.88,5.24 25.88,5.87 26.51,5.87 26.51,5.24 26.51,4.6 26.51,3.97 26.51,3.33 27.15,3.33 27.15,3.97 27.15,4.6 27.15,5.24 27.78,3.97 27.78,3.33 33.97,30.16 33.97,29.53 33.97,28.89 33.97,28.26 33.97,27.62 33.97,26.99 33.34,30.16 33.34,29.53 33.34,28.89 33.34,28.26 33.34,27.62 33.34,26.99 32.7,30.16 32.7,29.53 32.7,28.89 32.7,28.26 32.7,27.62 32.7,26.99 32.07,30.16 32.07,29.53 32.07,28.89 32.07,28.26 32.07,27.62 32.07,26.99 32.7,24.92 32.7,24.29 32.7,23.65 32.7,23.02 32.7,22.38 32.7,21.75 32.07,24.92 32.07,24.29 32.07,23.65 32.07,23.02 32.07,22.38 32.07,21.75 33.97,24.92 33.97,24.29 33.97,23.65 33.97,23.02 33.97,22.38 33.97,21.75 33.34,24.92 33.34,24.29 33.34,23.65 33.34,23.02 33.34,22.38 33.34,21.75 31.43,24.92 31.43,24.29 31.43,23.65 31.43,23.02 31.43,22.38 31.43,21.75 31.43,30.16 31.43,29.53 31.43,28.89 31.43,28.26 31.43,27.62 31.43,26.99 24.61,2.7 24.61,2.06 25.24,2.7 25.24,2.06 25.88,2.06 25.88,2.7 26.51,2.7 26.51,2.06 27.15,2.06 27.15,2.7 27.78,2.7 27.78,2.06 24.61,1.43 24.61,0.79 25.24,1.43 25.24,0.79 25.88,0.79 25.88,1.43 26.51,1.43 26.51,0.79 27.15,0.79 27.15,1.43 27.78,1.43 27.78,0.79 20.8,2.06 21.43,2.06 22.07,2.06 22.7,2.06 23.34,2.06 23.97,2.06 20.8,1.43 20.8,0.79 21.43,1.43 21.43,0.79 22.07,0.79 22.07,1.43 22.7,1.43 22.7,0.79 23.34,0.79 23.34,1.43 23.97,1.43 23.97,0.79 16.99,2.06 17.62,2.06 18.26,2.06 18.89,2.06 19.53,2.06 20.16,2.06 16.99,1.43 16.99,0.79 17.62,1.43 17.62,0.79 18.26,0.79 18.26,1.43 18.89,1.43 18.89,0.79 19.53,0.79 19.53,1.43 20.16,1.43 20.16,0.79 13.18,2.06 13.81,2.06 14.45,2.06 15.08,2.06 15.72,2.06 16.35,2.06 13.18,1.43 13.18,0.79 13.81,1.43 13.81,0.79 14.45,0.79 14.45,1.43 15.08,1.43 15.08,0.79 15.72,0.79 15.72,1.43 16.35,1.43 16.35,0.79 10.64,2.06 11.27,2.06 11.91,2.06 12.54,2.06 10.64,1.43 10.64,0.79 11.27,1.43 11.27,0.79 11.91,0.79 11.91,1.43 12.54,1.43 12.54,0.79 10.64,3.97 11.27,3.97 11.91,3.97 12.54,3.97 10.64,3.33 10.64,2.7 11.27,3.33 11.27,2.7 11.91,2.7 11.91,3.33 12.54,3.33 12.54,2.7 10.64,5.87 11.27,5.87 11.91,5.87 12.54,5.87 10.64,5.24 10.64,4.6 11.27,5.24 11.27,4.6 11.91,4.6 11.91,5.24 12.54,5.24 12.54,4.6 28.42,4.6 28.42,3.97 28.42,3.33 29.05,4.6 29.05,3.97 29.05,3.33 29.69,3.33 29.69,3.97 29.69,4.6 30.32,4.6 30.32,3.97 30.32,3.33 30.96,3.33 30.96,3.97 30.96,4.6 31.59,4.6 31.59,3.97 31.59,3.33 28.42,2.7 28.42,2.06 29.05,2.7 29.05,2.06 29.69,2.06 29.69,2.7 30.32,2.7 30.32,2.06 30.96,2.06 30.96,2.7 31.59,2.7 31.59,2.06 28.42,1.43 28.42,0.79 29.05,1.43 29.05,0.79 29.69,0.79 29.69,1.43 30.32,1.43 30.32,0.79 30.96,0.79 30.96,1.43 31.59,1.43 31.59,0.79 32.23,4.6 32.23,3.97 32.23,3.33 32.86,4.6 32.86,3.97 32.86,3.33 33.5,3.33 33.5,3.97 33.5,4.6 34.13,4.6 34.13,3.97 34.13,3.33 34.77,3.33 34.77,3.97 34.77,4.6 35.4,4.6 35.4,3.97 35.4,3.33 32.23,2.7 32.23,2.06 32.86,2.7 32.86,2.06 33.5,2.06 33.5,2.7 34.13,2.7 34.13,2.06 34.77,2.06 34.77,2.7 35.4,2.7 35.4,2.06 32.23,1.43 32.23,0.79 32.86,1.43 32.86,0.79 33.5,0.79 33.5,1.43 34.13,1.43 34.13,0.79 34.77,0.79 34.77,1.43 35.4,1.43 35.4,0.79 30.8,30.16 30.8,29.53 30.8,28.89 30.8,28.26 30.8,27.62 30.8,26.99 30.16,30.16 30.16,29.53 30.16,28.89 30.16,28.26 30.16,27.62 30.16,26.99 29.53,30.16 29.53,29.53 29.53,28.89 29.53,28.26 29.53,27.62 29.53,26.99 30.8,24.92 30.8,24.29 30.8,23.65 30.8,23.02 30.8,22.38 30.8,21.75 30.16,24.92 30.16,24.29 30.16,23.65 30.16,23.02 30.16,22.38 30.16,21.75 29.53,24.92 29.53,24.29 29.53,23.65 29.53,23.02 29.53,22.38 29.53,21.75 40.96,29.53 37.94,29.53 40.96,26.51 43.97,29.53 38.42,30 40.01,31.59 38.89,30.48 39.45,31.04 40.48,32.07 38.42,29.05 38.89,28.57 41.43,32.07 41.91,31.59 43.5,30 43.02,30.48 42.47,31.04 43.5,29.05 43.02,28.57 41.43,26.99 41.91,27.46 40.48,26.99 40.01,27.46 39.45,28.02 42.47,28.02 40.48,31.11 41.43,31.11 40.96,31.59 40.96,30.64 38.89,29.53 39.37,30 39.37,29.05 40.96,27.46 40.48,27.94 41.43,27.94 39.85,29.53 40.96,28.42 43.02,29.53 42.55,29.05 42.55,30 42.07,29.53 39.93,28.5 40.4,28.97 41.99,30.56 41.51,30.08 39.93,30.56 40.4,30.08 41.99,28.5 41.51,28.97 34.29,16.99 34.92,16.99 35.56,16.99 36.2,16.99 36.83,16.99 34.29,17.62 34.92,17.62 35.56,17.62 36.2,17.62 36.83,17.62 34.29,16.35 34.92,16.35 35.56,16.35 36.2,16.35 36.83,16.35 34.29,9.21 34.29,8.57 34.29,9.84 34.92,9.84 35.56,9.84 36.2,9.84 36.83,9.84 34.92,9.21 35.56,9.21 36.2,9.21 36.83,9.21 34.92,8.57 35.56,8.57 36.2,8.57 36.83,8.57
  pour Top (no thermals): 31.11,30.48 34.29,30.48 34.29,26.67 31.11,26.67
  pour Top (no thermals): 31.11,25.24 34.29,25.24 34.29,21.43 31.11,21.43
  pour Top (no thermals): 9.84,7.3 11.75,9.21 12.22,9.21 13.02,8.41 13.02,2.38 24.29,2.38 24.29,6.19 26.67,6.19 27.94,4.92 38.1,4.92 38.1,0.48 9.84,0.48
  pour Bottom (isolate 0.305, rank 3, no thermals): 0.32,40.48 0.32,0.48 38.1,0.48 38.1,23.18 44.45,29.53 38.1,35.88 38.1,40.48
CANH
  Top 0.406: IC2.7 54.93,9.84 57.52,7.25 R5.1 58.15,6.36 P3.1
CANL
  Top 0.406: IC2.6 54.77,8.57 55.82,7.52 R5.2 56.15,6.66 P3.2
CB
  Top 0.305: IC3.44 C13.1
CLK_MAG
  Top 0.203: IC1.10 43.73,16.83 41.59,16.83 40.48,15.72 40.48,5.89 P1.5
CPH
  Top 0.305: IC3.4 37.33,34.93 C45.2
CPL
  Top 0.305: IC3.3 38.26,34.7 38.26,35.88 37.31,36.83 C45.1
CS_MAG
  Top 0.203: IC1.9 42.91,17.31 42.91,17.3 42.07,17.3 | 42.07,17.3 41.43,17.3 40.01,15.88 40.01,4.37 P1.6 | RPULL2.2 42.12,17.36 42.07,17.3
DVDD
  Top 0.203: IC3.36 46.34,29.03 C14.1
ENABLE  (via drill 0.35)
  Top 0.203: IC3.38 45.41,30.8 46.04,30.8 48.42,33.18 48.74,33.18 49.21,33.66 49.21,34.29 48.74,34.77 47.94,34.77 | IC3.40 44.95,31.75 45.72,31.75 47.62,33.66 47.62,34.45 | IC3.42 44.49,32.7 45.4,32.7 46.04,33.34 46.04,34.29 46.51,34.77 47.31,34.77 | 47.31,34.77 47.62,34.45 | 47.94,34.77 47.78,34.77 | 47.78,34.77 47.62,34.77 | 47.62,34.77 47.47,34.77 | 47.47,34.77 47.31,34.77 | 47.62,34.45 47.62,34.61 47.78,34.77 | 47.62,34.45 47.94,34.77 | 47.62,34.77 47.62,34.92 | 47.62,34.92 v47.62,35.24 | 47.47,34.77 47.62,34.92 | 47.78,34.77 47.62,34.92 | IC1.13 42.45,15.31 v42.23,15.08
  Bottom 0.203: v47.62,35.24 46.99,35.24 46.04,34.29 46.04,33.5 46.83,32.7 46.83,21.27 44.77,19.21 44.77,15.88 43.97,15.08 v42.23,15.08
ENC_A  (via drill 0.35)
  Top 0.203: IC1.30 50.37,16.31 v50.8,15.88 | RPULL4.1 58.05,33.71 P2.3
  Bottom 0.305: v50.8,15.88 51.59,16.67 51.59,27.26 P2.3
ENC_B  (via drill 0.35)
  Top 0.203: IC1.29 49.6,15.81 v49.85,15.56 | RPULL3.1 58,35.66 P2.2
  Bottom 0.305: v49.85,15.56 49.85,16.19 50.96,17.3 50.96,28.62 P2.2
FB
  Top 0.305: IC3.1 40.16,34.21 40.16,35.08 | 40.16,35.08 40.16,35.4 | 40.48,35.4 40.9,35.4 R1.1 | 40.48,35.4 40.16,35.4 | 40.16,35.4 39.85,35.4 | 39.85,35.4 39.43,35.4 R2.2 | 40.48,35.4 40.16,35.08 | 40.16,35.08 39.85,35.4
FDCAN_RX
  Top 0.203: 47.93,7.3 48.26,7.3 | 48.26,7.3 IC2.4 | 48.26,7.3 47.62,6.67 45.72,6.67 45.4,6.99 45.4,10.16 45.72,10.48 46.83,10.48 47.15,10.79 47.15,11.75 46.45,12.45 IC1.21
FDCAN_TX
  Top 0.203: IC2.1 46.95,12.57 IC1.22
GAIN
  Top 0.203: IC3.32 44.72,26.83 46.67,26.83 R3.2
GHA
  Top 0.203: IC3.8 37.04,32.38 26.35,32.38 26.04,32.7 22.83,32.7 HAA.4
GHB
  Top 0.203: HBB.4 23.15,14.13 36.67,14.13 37.62,15.08 37.62,18.1 37.15,18.57 37.15,26.78 IC3.17
GHC
  Top 0.203: HCC.4 22.67,8.41 26.83,8.41 28.89,6.35 36.2,6.35 38.1,8.26 38.1,18.26 37.62,18.73 37.62,26.55 IC3.18
GLA
  Top 0.203: IC3.10 36.58,31.43 24.87,31.43 LAA.4
GLB  (via drill 0.35)
  Top 0.203: LBB.4 25.26,25.42 25.56,25.72 34.13,25.72 34.77,26.35 34.77,28.42 v35.88,29.53 | 37.26,28.32 IC3.15 36.2,27.24 36.2,25.08 v35.88,24.77
  Bottom 0.203: v35.88,29.53 v35.88,24.77
GLC
  Top 0.203: LCC.4 26.49,7.16 28.26,5.4 36.83,5.4 39.05,7.62 39.05,18.57 38.58,19.05 38.58,26.09 IC3.20
GND  (via drill 0.35)
  Top 0.203: R7.1 R10.1 50.53,31.22 50.9,31.59 R6.1 50.9,33.23 v52.28,34.61 | IC3.35 45.41,28.26 46.83,28.26 47.86,29.29 | C14.2 49.05,31.05 49.05,30.48 48.18,29.61 | 47.86,29.29 48.02,29.45 | 48.02,29.45 48.18,29.61 | IC3.27 44.2,23.81 C15.2 | XT1.2 48.1,20.95 v49.05,21.91 | C27.2 46.93,9.84 IC2.2 | C4.1 44.19,6.35 44.66,5.87 48.5,5.87 P1.1 52.62,1.75 58.9,1.75 59.53,2.38 59.53,6.99 58.2,8.31 R11.1 | IC1.32 48.65,17.25 | IC1.31 IC1.32 | IC1.32 v49.53,17.3 50.43,17.3 C26.2 | 53.12,21.91 U$3.4 | 48.18,29.29 48.61,28.86 R3.1 48.7,29.18 v49.21,29.69 | 48.02,29.45 48.18,29.29 | 48.18,29.29 48.18,29.61 | 48.18,29.29 47.86,29.29 | IC1.16 43.02,13.08 v43.02,13.02
  Top 0.305: D1.2 46.76,39.21 v45.4,39.21 | 44.98,39 v44.77,39.21 | IC3.43 44.57,33.5 v45.09,33.5 45.09,33.55 | C14.2 50.36,31.4 50.53,31.22
  Top 0.406: R8.1 38.97,39.29 v39.05,39.21 | CIN.2 CIN1.2 44.98,39
  Bottom 0.203: v49.05,21.91 49.53,21.43 v49.53,17.3 | C15.2 43.81,23.28 C1.2 | C2.2 40.01,23.34 46.04,29.37 46.04,32.54 v45.09,33.5 | U$3.4 53.5,27.16 P2.4 | C27.2 51.2,4.74 P1.1
  Bottom 0.305: v45.4,39.21 49.69,39.21 | v52.28,34.61 52.28,36.62 49.69,39.21 | 49.69,39.21 50.48,40.01 59.69,40.01 60.64,39.05 60.64,33.81 59.23,32.4 P2.4
  Bottom 0.406: CIN.2 45.09,36.41 v45.09,33.5
  other vias: 39.37,37.05 39.05,39.85 39.69,39.85 39.69,39.21 40.32,39.85 40.32,39.21 40.96,39.21 40.96,39.85 41.59,39.85 41.59,39.21 42.23,39.85 42.23,39.21 42.86,39.21 42.86,39.85 43.5,39.85 43.5,39.21 44.13,39.21 44.13,39.85 44.77,39.85 45.4,39.85 44.98,36.51 44.35,23.81 40.01,19.95 43.81,19.95 53.5,21.53 46.51,9.42
  pour Top (no thermals): 33.81,40.16 33.81,38.89 45.72,38.89 45.72,40.16
  pour Bottom (isolate 0.305, no thermals): 38.73,40.32 38.73,36.2 45.4,29.53 38.73,22.86 38.73,0.48 61.91,0.48 61.91,40.32
IDRIVE
  Top 0.203: IC3.30 44.26,25.88 47.62,25.88 50.32,28.57 51.17,28.57 R7.2
LEDFAULT
  Top 0.203: RPULL1.2 51.44,27.46 52.55,27.46 53.98,28.89 LED1.1
LP_SOA
  Top 0.254: R12.1 45.95,19.24 IC1.5
LP_SOB
  Top 0.254: IC1.6 45.45,18.69 45.24,18.89 43.02,18.89 41.97,19.95 R13.1
MISO_MAG
  Top 0.203: IC1.11 41.71,16.31 40.96,15.56 40.96,6.03 42.55,4.45 43.93,4.45 P1.4
MODE
  Top 0.203: IC3.29 44.02,25.4 47.78,25.4 50.48,28.1 52.39,28.1 53.02,28.73 53.02,32.44 R6.2
MOSI_MAG
  Top 0.203: IC1.12 41.84,15.81 41.43,15.4 41.43,6.19 42.7,4.92 45.45,4.92 P1.3
N$9
  Top 0.203: IC1.3 46.95,20.12 XT1.3
N$10
  Top 0.203: R11.2 59.91,10.59 LED3.1
N$11
  Top 0.203: IC1.2 47.45,18.55 47.78,18.89 48.9,18.89 49.3,19.3 XT1.1
NFAULT
  Top 0.203: IC3.28 43.79,24.92 48.42,24.92 | RPULL1.1 48.9,24.92 | 48.42,24.92 48.58,24.92 | 48.58,24.92 48.9,24.92 | 48.9,24.92 48.58,24.61 | 48.58,24.61 47.78,23.81 RPULL.1 | 48.58,24.77 48.58,24.92 | 48.42,24.92 48.58,24.77 | 48.58,24.77 48.58,24.61
PHASEA
  Top 0.203: LAA.9 21.56,31.09 22.7,32.23 25.88,32.23 26.19,31.91 36.81,31.91 IC3.9
  pour Top (isolate 0.203, no thermals): 22.54,34.61 20.64,34.61 20.64,33.02 23.34,30.32 23.34,26.83 18.73,26.83 17.14,25.24 9.84,25.24 9.84,31.11 12.54,31.11 13.65,32.23 13.65,37.94 22.54,37.94
PHASEB
  Top 0.203: LBB.8 20.56,20.16 34.77,20.16 36.67,22.07 36.67,27.01 IC3.16
  pour Top (isolate 0.203, no thermals): 23.34,26.19 23.34,20.32 22.54,20.32 22.54,16.35 9.84,16.35 9.84,24.61 17.3,24.61 18.89,26.19
PHASEC
  Top 0.203: LCC.9 21.56,5.84 23.65,7.94 26.51,7.94 28.57,5.87 36.51,5.87 38.58,7.94 38.58,18.41 38.1,18.89 38.1,26.32 IC3.19
  pour Top (isolate 0.203, no thermals): 22.54,13.89 21.51,13.89 19.68,15.72 9.84,15.72 9.84,9.84 12.54,9.84 13.65,8.73 13.65,3.02 23.34,3.02 23.34,5.71 20.64,8.41 20.64,10.16 22.54,10.16
PWMA  (via drill 0.35)
  Top 0.203: IC3.37 45.64,30.32 46.2,30.32 48.58,32.7 49.37,32.7 v49.69,33.02 | v46.51,11.27 45.95,11.84 IC1.20
  Bottom 0.203: v49.69,33.02 48.26,31.59 48.26,20.32 46.2,18.26 46.2,11.59 v46.51,11.27
PWMB  (via drill 0.35)
  Top 0.203: IC3.39 45.18,31.27 45.88,31.27 48.42,33.81 v48.42,33.97 | IC1.19 45.45,11.31 v45.4,11.27
  Bottom 0.203: v45.4,11.27 45.72,11.59 45.72,18.57 47.78,20.64 47.78,33.34 v48.42,33.97
PWMC  (via drill 0.35)
  Top 0.203: IC3.41 44.72,32.23 45.56,32.23 46.83,33.5 v46.83,33.97 | v44.61,11.91 44.95,12.24 IC1.18
  Bottom 0.203: v46.83,33.97 47.31,33.5 47.31,20.95 45.24,18.89 45.24,12.54 v44.61,11.91
SOA
  Top 0.305: IC3.25 40.82,24.51 40.82,23.95 43.12,21.65 C1.1 R12.2
SOB
  Top 0.305: IC3.24 40.01,24.69 C2.1 R13.2
SPA  (via drill 0.35)
  Top 0.203: R14.2 27.74,29.8 28.89,30.96 36.35,30.96 IC3.11
  other vias: 24.61,30.16 24.61,29.53 25.24,29.53 24.61,28.89 24.61,28.26 24.61,27.62 25.24,30.16 25.24,28.89 25.24,28.26 25.24,27.62 27.46,30.16 27.46,29.53 28.1,29.53 27.46,28.89 27.46,28.26 27.46,27.62 28.1,30.16 28.1,28.89 28.1,28.26 28.1,27.62 24.61,26.99 25.24,26.99 28.1,26.99 27.46,26.99 25.88,30.16 25.88,29.53 25.88,28.89 25.88,28.26 25.88,27.62 25.88,26.99 26.83,26.99 26.83,27.62 26.83,28.26 26.83,28.89 26.83,29.53 26.83,30.16
  pour Top (isolate 0.203, no thermals): 24.29,30.48 28.42,30.48 28.42,26.19 24.29,26.19
  pour Bottom (isolate 0.203, no thermals): 24.29,26.19 24.29,30.48 28.42,30.48 28.42,26.19
SPB  (via drill 0.35)
  Top 0.203: IC3.14 35.72,27.47 35.72,25.72 34.92,24.92 34.92,21.43 34.45,20.95 v28.1,20.95
  other vias: 24.61,24.13 24.61,23.5 24.61,22.86 24.61,22.23 24.61,21.59 24.61,20.95 25.24,24.13 25.24,23.5 25.24,22.86 25.24,22.23 25.24,21.59 27.46,24.77 28.1,24.13 27.46,24.13 27.46,23.5 28.1,23.5 28.1,22.86 27.46,22.86 28.1,22.23 27.46,22.23 28.1,21.59 27.46,21.59 27.46,20.95 25.24,20.95 28.1,24.77 25.88,24.13 25.88,23.5 25.88,22.86 25.88,22.23 25.88,21.59 25.88,20.95 26.83,20.95 26.83,21.59 26.83,22.23 26.83,22.86 26.83,23.5 26.83,24.13 26.83,24.77
  pour Top (isolate 0.203, no thermals): 24.29,24.45 24.29,20.64 28.42,20.64 28.42,25.08 26.67,25.08 26.04,24.45
  pour Bottom (isolate 0.203, no thermals): 24.29,24.45 26.04,24.45 26.67,25.08 28.42,25.08 28.42,20.64 24.29,20.64
SW
  Top 0.305: IC3.45 43.28,33.62 C13.2 43.28,35.19 43.66,35.56 46.11,35.56 D1.1 47.15,37.31 49.39,39.55 L2.1
SWCLK
  Top 0.203: IC1.24 48.04,13.02 49.05,13.02 50.48,14.45 55.56,14.45 55.88,14.76 55.88,16.51 54.86,17.53 U$3.2
SWIO
  Top 0.203: IC1.23 47.47,13.09 47.47,12.54 47.62,12.38 49.21,12.38 50.8,13.97 55.88,13.97 56.36,14.45 56.36,18.1 54.93,19.53 U$3.3
SWO
  Top 0.203: IC1.26 49.55,14.31 50.16,14.92 51.47,14.92 52.07,15.53 U$3.1
VCP
  Top 0.305: C11.2 35.4,33.76 37.79,33.76 IC3.5
VDS
  Top 0.203: IC3.31 44.49,26.35 47.47,26.35 50.48,29.37 R10.2

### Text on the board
tPlace: 3V3 | B | A | VIN | GND | FAULT | U | 3V3 | GND | V | IO | CLK | O | W | POWER | GND | CS | CLK | MI | MO | 3V3 | GND | CANL | CANH

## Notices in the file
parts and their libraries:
SparkFun-Coils: Licensing: Creative Commons ShareAlike 4.0 International - https://creativecommons.org/licenses/by-sa/4.0
